(* Generated automatically by TwinCAT - (read only) *)
VAR_CONFIG
	FAST.iCounter AT %QB0 : UDINT;	(*  ~ {LinkedWith:TIID^Device 2 (EtherCAT)^Term 1 (CX1100-0004)^Term 2 (EK1122)^Term 3 (EK1101)^Term 4 (EL2002)^Channel 1^Output;TIID^Device 2 (EtherCAT)^Term 1 (CX1100-0004)^Term 2 (EK1122)^Term 3 (EK1101)^Term 4 (EL2002)^Channel 2^Output} *)
	FAST.iTest AT %IB24 : UDINT;
	FAST.wFrmXWcState AT %IB0 : WORD;	(*  ~ {LinkedWith:TIID^Device 2 (EtherCAT)^Inputs^Frm0WcState} *)
	MAIN.iCounter AT %QB4 : UDINT;	(*  ~ {LinkedWith:TIID^Device 2 (EtherCAT)^Term 1 (CX1100-0004)^Term 2 (EK1122)^Term 3 (EK1101)^Term 5 (EL2032)^Channel 1^Output;TIID^Device 2 (EtherCAT)^Term 1 (CX1100-0004)^Term 2 (EK1122)^Term 3 (EK1101)^Term 5 (EL2032)^Channel 2^Output;TIID^Device 1 (EL6731)^Box 11  (BK3150)^Term 2 (KL2114)^Channel 1^Output;TIID^Device 1 (EL6731)^Box 11  (BK3150)^Term 2 (KL2114)^Channel 2^Output;TIID^Device 1 (EL6731)^Box 11  (BK3150)^Term 2 (KL2114)^Channel 3^Output;TIID^Device 1 (EL6731)^Box 11  (BK3150)^Term 2 (KL2114)^Channel 4^Output;TIID^Device 1 (EL6731)^Box 14  (BK3120)^Term 6 (KL2012)^Channel 1^Output;TIID^Device 1 (EL6731)^Box 14  (BK3120)^Term 6 (KL2012)^Channel 2^Output;TIID^Device 1 (EL6731)^Box 31  (BK3110)^Term 11 (KL2114)^Channel 1^Output;TIID^Device 1 (EL6731)^Box 31  (BK3110)^Term 11 (KL2114)^Channel 2^Output;TIID^Device 1 (EL6731)^Box 31  (BK3110)^Term 11 (KL2114)^Channel 3^Output;TIID^Device 1 (EL6731)^Box 31  (BK3110)^Term 11 (KL2114)^Channel 4^Output} *)
	MAIN.iTest AT %IB20 : UDINT;	(*  ~ {LinkedWith:TIID^Device 2 (EtherCAT)^Term 1 (CX1100-0004)^Box 23 (BK1250)^Term 13 (KL1408)^Channel 1^Input;TIID^Device 2 (EtherCAT)^Term 1 (CX1100-0004)^Box 23 (BK1250)^Term 13 (KL1408)^Channel 2^Input;TIID^Device 2 (EtherCAT)^Term 1 (CX1100-0004)^Box 23 (BK1250)^Term 13 (KL1408)^Channel 3^Input;TIID^Device 2 (EtherCAT)^Term 1 (CX1100-0004)^Box 23 (BK1250)^Term 13 (KL1408)^Channel 4^Input;TIID^Device 2 (EtherCAT)^Term 1 (CX1100-0004)^Box 23 (BK1250)^Term 13 (KL1408)^Channel 5^Input;TIID^Device 2 (EtherCAT)^Term 1 (CX1100-0004)^Box 23 (BK1250)^Term 13 (KL1408)^Channel 6^Input;TIID^Device 2 (EtherCAT)^Term 1 (CX1100-0004)^Box 23 (BK1250)^Term 13 (KL1408)^Channel 7^Input;TIID^Device 2 (EtherCAT)^Term 1 (CX1100-0004)^Box 23 (BK1250)^Term 13 (KL1408)^Channel 8^Input} *)
	MAIN.wFrmXWcState AT %IB2 : WORD;	(*  ~ {LinkedWith:TIID^Device 2 (EtherCAT)^Inputs^Frm1WcState} *)
	MAIN.nEcMasterDeviceId AT %IB4 : UINT;	(*  ~ {LinkedWith:TIID^Device 2 (EtherCAT)^InfoData^DevId} *)
	MAIN.nEcMasterSlaveCount AT %IB6 : UINT;	(*  ~ {LinkedWith:TIID^Device 2 (EtherCAT)^Inputs^SlaveCount} *)
	MAIN.nEcMasterDevState AT %IB8 : UINT;	(*  ~ {LinkedWith:TIID^Device 2 (EtherCAT)^Inputs^DevState} *)
	MAIN.arrEcMasterNetId AT %IB10 : T_AmsNetIdArr;	(*  ~ {LinkedWith:TIID^Device 2 (EtherCAT)^InfoData^AmsNetId} *)
	MAIN.nEcMasterSlaveCountCfg AT %IB16 : UINT;	(*  ~ {LinkedWith:TIID^Device 2 (EtherCAT)^InfoData^CfgSlaveCount} *)
END_VAR
